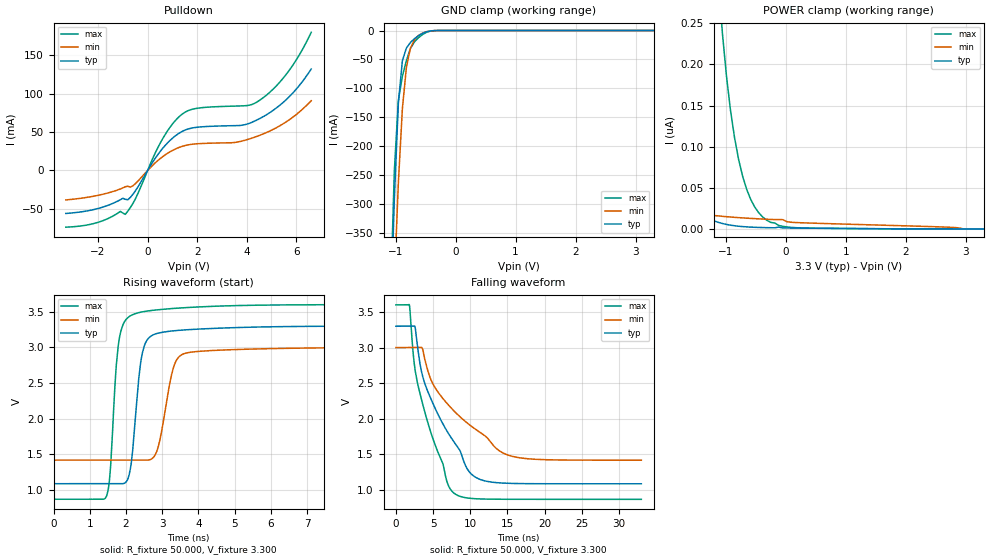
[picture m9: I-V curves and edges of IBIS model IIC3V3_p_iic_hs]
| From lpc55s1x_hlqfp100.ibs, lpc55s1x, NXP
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|   Model IIC3V3_p_iic_hs
[Model] IIC3V3_p_iic_hs
Model_type I/O_open_drain
Polarity   Non-Inverting
Enable   Active-Low
Vinl =  0.990V
Vinh =  2.310V
Vmeas =  1.650V
Cref =  0.0F
Rref =  100.000
Vref =  3.3V
C_comp   2.333pF   2.290pF   2.366pF
C_comp_pulldown   1.603pF   1.542pF   1.653pF
C_comp_power_clamp   0.444pF   0.380pF   0.497pF
[Model Spec]
Vinh   2.310V   2.100V   2.520V
Vinl   0.990V   0.900V   1.080V
Vmeas   1.650V   1.500V   1.800V
Vref   3.3V   3.0V   3.6V
Cref   0.0F   0.0F   0.0F
Rref   100.000   100.000   100.000
[Temperature Range]   25.000   0.125k   -40.000
[Voltage Range]   3.300V   3.000V   3.600V
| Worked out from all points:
|   slope of the pulldown table from 0 to 0.495 V, typ, clamps not added: 20.4 ohm
|   GND clamp passes 1 mA (typ) near -0.43 V on its own axis
|   rising waveform, R_fixture 50.000, V_fixture 3.300: 20-80 % time 248ps typ, 344ps min, 210ps max; typ from 1.08 V to 3.3 V
|   falling waveform, R_fixture 50.000, V_fixture 3.300: 20-80 % time 5.6ns typ, 8ns min, 3.92ns max; typ from 3.3 V to 1.08 V
[Pulldown]
|Voltage   I(typ)   I(min)   I(max)
-3.3V     -56mA      -38.4mA    -73.87mA
-2.1V     -50.37mA   -33.07mA   -68.52mA
-1.1V     -38.15mA   -24.11mA   -53.37mA
-900mV    -37.61mA   -21.16mA   -57.18mA
-500mV    -26.92mA   -17.4mA    -37.43mA
500mV     24.51mA    15.34mA    35.14mA
1.2V      47.07mA    29.16mA    67.89mA
1.9V      55.94mA    34.55mA    80.54mA
3.8V      58.94mA    38.34mA    84.23mA
4.5V      67.28mA    45.58mA    91.12mA
5.6V      92.63mA    63.59mA    125.7mA
6.6V      132.3mA    90.99mA    180.1mA
[GND_clamp]
|Voltage   I(typ)   I(min)   I(max)
-3.3V     -10.05A    -9.18A     -11.33A
-1.089V   -516.5mA   -633.7mA   -475mA
-1.022V   -291.8mA   -436.3mA   -243.2mA
-955mV    -126mA     -264mA     -120.7mA
-888mV    -52.17mA   -135.6mA   -79.11mA
-821mV    -30.43mA   -63.68mA   -52.11mA
-754mV    -20.66mA   -30.68mA   -31.04mA
-687mV    -14.18mA   -15.96mA   -19.64mA
-553mV    -5.013mA   -4.505mA   -7.034mA
-419mV    -652.2uA   -708.2uA   -887.6uA
-285mV    -14.83uA   -32.68uA   -16.3uA
3.3V      0A         0A         0A
[POWER_clamp]
|Voltage   I(typ)   I(min)   I(max)
-3.3V     1.337uA    96.84nA    41.74uA
-2.395V   241.1nA    38.51nA    8.841uA
-2.194V   152.2nA    32.17nA    5.805uA
-1.926V   78.16nA    25.86nA    3.134uA
-1.658V   37.82nA    21.36nA    1.572uA
-1.256V   11.75nA    16.9nA     472.7nA
-1.055V   6.592nA    15.36nA    237.1nA
-921mV    4.605nA    14.51nA    144.1nA
-787mV    3.339nA    13.77nA    84.89nA
-586mV    2.257nA    12.84nA    36.19nA
-318mV    1.588nA    11.83nA    10.67nA
3.3V      0A         0A         0A
[Ramp]
| variable   typ   min   max
dV/dt_r   1.329/0.248n   0.950/0.343n   1.640/0.209n
dV/dt_f   1.329/5.600n   0.950/7.994n   1.640/3.921n
R_load = 50.000
[Rising Waveform]
R_fixture= 50.000
V_fixture= 3.300
V_fixture_min= 3.000
V_fixture_max= 3.600
|time   V(typ)   V(min)   V(max)
0s        1.085V     1.416V     866.9mV
1.467ns   1.085V     1.416V     916.2mV
1.566ns   1.085V     1.416V     1.26V
1.774ns   1.085V     1.416V     2.969V
2.027ns   1.126V     1.416V     3.404V
2.508ns   3.022V     1.415V     3.502V
2.881ns   3.197V     1.586V     3.526V
3.376ns   3.234V     2.8V       3.547V
3.895ns   3.252V     2.937V     3.563V
33ns      3.3V       3V         3.6V
[Falling Waveform]
R_fixture= 50.000
V_fixture= 3.300
V_fixture_min= 3.000
V_fixture_max= 3.600
|time   V(typ)   V(min)   V(max)
0s        3.3V       3V         3.6V
1.806ns   3.3V       3V         3.599V
2.551ns   3.295V     3V         2.705V
3.004ns   2.938V     3V         2.453V
4.258ns   2.389V     2.685V     1.955V
7.777ns   1.679V     2.113V     956.2mV
9.917ns   1.247V     1.912V     882mV
12.01ns   1.125V     1.757V     870.3mV
16.64ns   1.088V     1.451V     867.2mV
33ns      1.085V     1.416V     866.9mV
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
